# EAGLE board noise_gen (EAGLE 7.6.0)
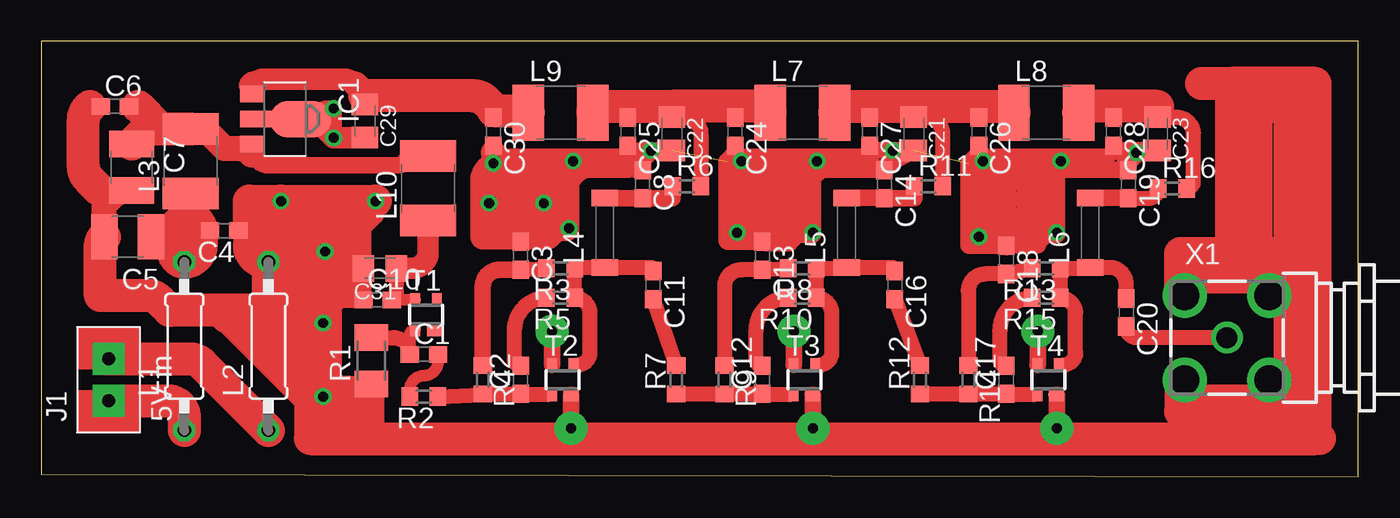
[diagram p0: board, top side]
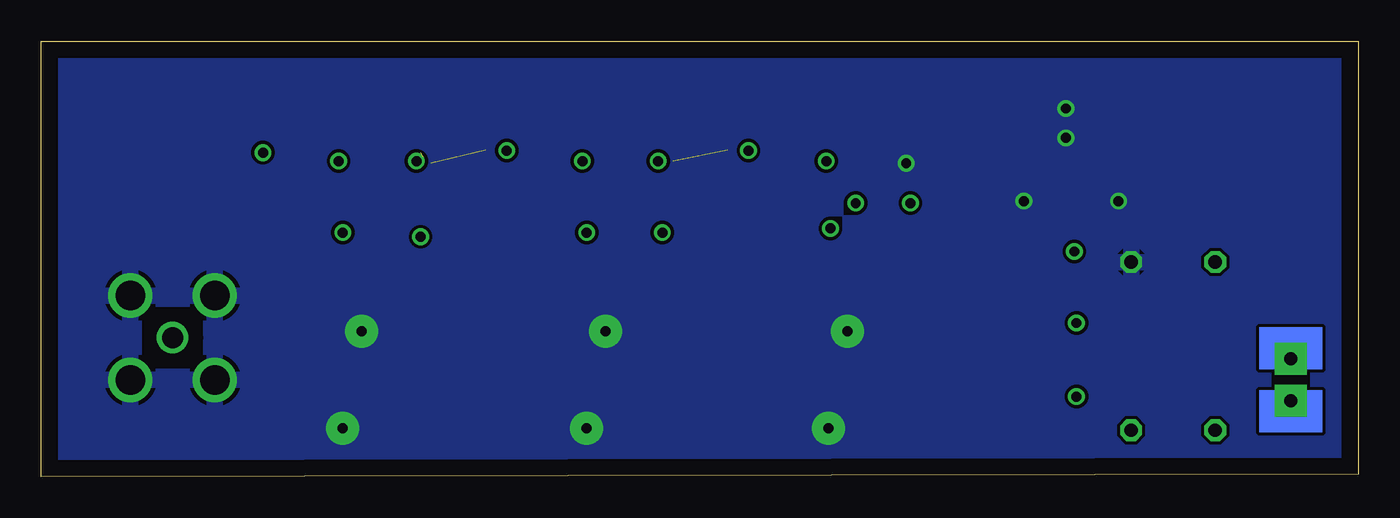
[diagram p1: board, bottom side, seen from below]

Size 79.55 x 26.28 mm. Coordinates in mm from the lower left corner, seen from the top.
Outline: 0,0.13 79.55,0 79.55,26.28 0,26.28 0,0.13
Copper layers (1*16): Top 0.035mm / dielectric 1.5mm / Bottom 0.035mm
Design rules "default": minimum track width 10mil, minimum drill 24mil, track to track 8mil, track to pad 8mil, pad to pad 8mil, via to via 8mil, smd to smd 8mil, copper to edge 40mil, drill to drill 8mil, minimum pad ring 10mil, minimum via ring 8mil, stop-mask expansion 4mil, vias tented up to drill 0mil, thermal gap 10mil

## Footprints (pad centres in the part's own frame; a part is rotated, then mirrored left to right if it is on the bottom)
C0603 = smd 1.1 x 1: 1 -0.85,0; 2 0.85,0
C1210 = smd 1.6 x 2.7: 1 -1.4,0; 2 1.4,0
C0805K = smd 1.3 x 1.6: 1 -1,0; 2 1,0
SOT89 = smd 1 x 1.5: 1 -1.499,-1.981; 3 1.499,-1.981 | smd 1 x 2: 2 0,-1.727 | smd 2.2 x 3.7: 2@1 0,0.94
H2-2.54_BIIG = drill 0.8 pad 1.93 square: 1 0,0; 2 0,2.54
0207/10 = drill 0.813 octagon: 1 -5.08,0; 2 5.08,0
L1812 = smd 1.9 x 3.4: 1 -1.95,0; 2 1.95,0
L4516C = smd 1 x 1.6: 1 -2.1,0; 2 2.1,0
M1206 = smd 1.6 x 2: 1 -1.4,0; 2 1.4,0
R0603 = smd 1 x 1.1: 1 -0.85,0; 2 0.85,0
SOT343R = smd 0.9 x 0.8: 1 0.5,-0.9 | smd 0.6 x 0.8: 2 -0.65,-0.9; 3 -0.65,0.9; 4 0.65,0.9
BU-SMA-G = drill 1.27: 1 0,0 | drill 1.778: 2 -2.55,2.55; 3 2.55,2.55; 4 2.55,-2.55; 5 -2.55,-2.55

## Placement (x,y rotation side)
C1  1n  [C0603]  23.11,7.37 0 top
C2  1n  [C0603]  28.96,5.84 90 top
C3  1n  [C0603]  28.96,13.34 270 top
C4  1 nF  [C0603]  11.05,14.86 180 top
C5  10 uF  [C1210]  5.21,14.48 180 top
C6  1 nF  [C0603]  4.45,22.35 0 top
C7  10 uF  [C1210]  5.46,18.67 270 top
C8  3n3  [C0603]  36.32,17.65 270 top
C10  3n3  [C0603]  20.32,10.67 0 top
C11  1n  [C0603]  36.96,11.56 270 top
C12  1n  [C0603]  43.56,5.84 90 top
C13  1n  [C0603]  43.56,13.34 270 top
C14  3n3  [C0603]  50.93,17.65 270 top
C16  1n  [C0603]  51.56,11.56 270 top
C17  1n  [C0603]  58.29,5.84 90 top
C18  1n  [C0603]  58.29,13.08 270 top
C19  3n3  [C0603]  65.66,17.65 270 top
C20  [C0603]  65.53,9.91 270 top
C21  100nF  [C0805K]  52.7,20.7 270 top
C22  100nF  [C0805K]  38.1,20.7 270 top
C23  100nF  [C0805K]  67.44,20.7 270 top
C24  1 nF  [C0603]  41.91,20.83 270 top
C25  1 nF  [C0603]  35.43,20.83 270 top
C26  1 nF  [C0603]  56.64,20.83 270 top
C27  1 nF  [C0603]  50.04,20.83 270 top
C28  1 nF  [C0603]  64.77,20.83 270 top
C29  100nF  [C0805K]  19.56,21.46 270 top
C30  1 nF  [C0603]  27.3,20.83 270 top
C31  100nF  [C0805K]  20.45,12.57 180 top
IC1  78L3.3F  [SOT89]  14.73,21.59 270 top
J1  5V in  [H2-2.54_BIIG]  4.06,4.57 0 top
L1  [0207/10]  8.64,7.87 90 top
L2  [0207/10]  13.72,7.87 90 top
L3  [L1812]  9.02,19.05 90 top
L4  60 nH  [L4516C]  34.04,14.73 90 top
L5  60 nH  [L4516C]  48.64,14.73 90 top
L6  60 nH  [L4516C]  63.37,14.73 90 top
L7  [L1812]  45.97,21.97 0 top
L8  [L1812]  60.71,21.97 0 top
L9  [L1812]  31.37,21.97 0 top
L10  [L1812]  23.37,17.4 90 top
R1  1k5  [M1206]  19.94,6.98 90 top
R2  18  [R0603]  23.11,4.83 180 top
R3  1k5  [R0603]  31.37,12.57 180 top
R4  1k5  [R0603]  26.67,5.84 270 top
R5  510R  [R0603]  31.37,10.79 180 top
R6  100  [R0603]  38.99,17.53 0 top
R7  18  [R0603]  38.35,5.84 90 top
R8  1k5  [R0603]  45.97,12.57 180 top
R9  1k5  [R0603]  41.27,5.84 270 top
R10  510R  [R0603]  45.97,10.79 180 top
R11  100  [R0603]  53.59,17.53 0 top
R12  18  [R0603]  53.09,5.84 90 top
R13  1k5  [R0603]  60.71,12.57 180 top
R14  1k5  [R0603]  56.01,5.84 270 top
R15  510R  [R0603]  60.71,10.79 180 top
R16  100  [R0603]  68.33,17.4 0 top
T1  BFG425W  [SOT343R]  23.24,9.78 0 top
T2  BFG425W  [SOT343R]  31.5,5.84 0 top
T3  BFG425W  [SOT343R]  46.1,5.84 0 top
T4  BFG425W  [SOT343R]  60.83,5.84 0 top
X1  BU-SMA-G  [BU-SMA-G]  71.63,8.38 0 top

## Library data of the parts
C1-C8 C10-C14 C16-C31 L1-L10 R1-R16 = rcl
IC1 = linear
J1 = Seeed-OPL-Connector
T1-T4 = mylib
X1 = con-coax; OC_FARNELL: unknown; OC_NEWARK: unknown

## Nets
GND: C3.1 C4.1 C5.2 C6.1 C7.2 C8.1 C10.1 C13.1 C14.1 C18.1 C19.1 C21.2 C22.2 C23.2 C24.2 C25.2 C26.2 C27.2 C28.2 C29.2 C30.2 C31.2 IC1.2 IC1.2@1 L2.2 R1.1 T2.1 T2.3 T3.1 T3.3 T4.1 T4.3 X1.2 X1.3 X1.4 X1.5
N$1: C29.1 C30.1 IC1.1 L9.1
N$2: C1.2 R2.2
N$3: C2.1 R2.1 R4.2 T2.2
N$4: C3.2 R3.2 R4.1
N$5: C2.2 R5.2
N$6: C11.1 L4.1 R3.1 R5.1 T2.4
N$7: J1.1 L1.1
N$8: C4.2 C5.1 L1.2 L3.1
N$9: J1.2 L2.1
N$10: C6.2 C7.1 IC1.3 L3.2 L10.2
N$11: C8.2 L4.2 R6.1
N$12: C1.1 R1.2 T1.2
N$13: C10.2 C31.1 L10.1 T1.3
N$14: C11.2 R7.2
N$15: C12.1 R7.1 R9.2 T3.2
N$16: C13.2 R8.2 R9.1
N$17: C12.2 R10.2
N$19: C14.2 L5.2 R11.1
N$20: C16.2 R12.2
N$21: C17.1 R12.1 R14.2 T4.2
N$22: C18.2 R13.2 R14.1
N$23: C17.2 R15.2
N$24: C20.1 L6.1 R13.1 R15.1 T4.4
N$25: C19.2 L6.2 R16.1
N$27: C16.1 L5.1 R8.1 R10.1 T3.4
N$28: C20.2 X1.1
N$32: C22.1 C24.1 C25.1 L7.1 L9.2 R6.2
N$34: C21.1 C26.1 C27.1 L7.2 L8.1 R11.2
N$35: C23.1 C28.1 L8.2 R16.2

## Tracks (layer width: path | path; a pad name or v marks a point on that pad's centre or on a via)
GND  (via drill 0.6 pad 1, 0.6 pad 2)  (3 unrouted)
  Top 0.406: T2.1
  Top 0.9: C6.1 2.92,22.35 | C19.1 65.66,18.54 65.66,18.92 | C28.2 64.77,19.68 64.77,19.56 | 50.04,19.68 50.04,19.56 | C26.2 56.64,19.56 | C24.2 41.91,19.56 | C25.2 35.43,19.56 | C8.1 36.32,18.92 | C30.2 27.3,19.56 | C31.2 arc-90 19.47,12.55 C10.1 | IC1.2 IC1.2@1 | C4.1 12.57,14.86
  Top 1: T2.3 30.86,6.74 v30.86,8.76 | T2.1 v32,2.92 | T3.3 arc90 45.47,6.76 v45.47,8.76 | T3.1 arc-90 T3.1 v46.61,2.92 | T4.3 arc90 60.2,6.76 v60.2,8.76 | T4.1 arc-90 61.34,4.93 v61.34,2.92 | 36.32,18.92 arc-90 35.43,19.81 C25.2 | C14.1 arc-90 50.04,19.39 50.04,19.68 | 50.04,19.68 C27.2 arc90 50.31,19.7 C21.2 50.55,18.54 | 35.56,19.68 C22.2 37.32,19.7 arc90 36.32,18.7 C8.1 36.14,18.5 arc-45 35.43,18.8 | 65.66,18.92 66.14,19.41 arc-45 66.85,19.7 C23.2 65.44,19.7 arc-45 C28.2 65.37,19.38 arc-45 65.66,18.67 65.66,18.54 | 35.43,18.8 | C3.1 28.96,14.48 | C10.1 18.03,10.67 17.65,10.29 17.65,5.97 18.04,5.58 R1.1 | C31.2 19.43,12.59 19.43,14.99 20.19,15.75 v20.19,16.64 | 11.39,9.56 11.86,10.03 12.45,10.03 | 41.91,19.56 41.66,19.3 | 41.66,19.3 41.4,19.05 41.4,14.22 41.44,14.19 C13.1 | 56.64,19.56 56.01,18.92 56.01,13.97 56.05,13.93 C18.1 | 74.68,13.46 74.55,13.46 74.3,13.72 73.41,13.72 | 75.44,3.43 74.93,3.94 74.55,3.94 | 64.77,19.68 64.39,19.3 56.52,19.3 | 50.04,19.68 49.66,19.3 41.66,19.3 | 16.76,21.84 17.14,22.22 v17.65,22.22 v17.65,20.45
  Top 1.3: C29.2 17.69,20.46 arc45 v17.65,20.45 16.8,21.3 arc45 16.1,21.59 IC1.2@1
  Top 1.5: C5.2 arc45 C5.2 3.81,16.38 4.4,16.98 arc-45 5.11,17.27 C7.2 arc45 C7.2 3.56,17.27 | 27.3,19.56 v27.3,18.92 26.96,18.58 arc45 26.67,17.87 26.67,14.48 28.96,14.48 30.61,14.48 30.82,14.69 arc-45 31.53,14.99 31.75,14.99 31.75,17.91 32.35,18.5 arc-45 33.05,18.8 35.43,18.8
  Top 2: 3.56,17.27 2.83,17.99 arc-45 2.54,18.7 2.54,21.56 arc-45 2.83,22.26 2.92,22.35 | C5.2 arc45 3.56,13.87 3.56,10.92 6.44,10.92 arc-45 7.15,10.63 7.75,10.03 12.45,10.03 12.72,10.03 arc90 13.72,11.03 L2.2 13.57,12.95 arc-90 12.57,13.95 12.57,14.86 12.57,16.64 v14.48,16.64 v20.19,16.64 | 11.18,9.65 arc-45 11.39,9.56 16.26,4.7 16.26,2.29 32,2.29 | 32,2.29 v32,2.92 | X1.2 68.83,11.18 68.83,13.46 74.55,13.46 74.55,11.3 X1.3 | X1.5 68.83,5.59 68.83,3.94 74.55,3.94 74.55,5.46 X1.4 | 32,2.29 46.61,2.29 | 46.61,2.29 v46.61,2.92 | 46.61,2.29 61.34,2.29 | 61.34,2.29 v61.34,2.92 | 61.34,2.29 76.96,2.29 | 77.22,2.29 76.96,2.29 | 76.96,2.29 76.96,23.75 71.88,23.75 | 70.1,23.75 71.88,23.75 | 71.88,23.75 71.88,13.72 73.41,13.72 73.41,22.35 75.31,22.35 75.31,22.22 75.44,22.22 75.44,3.43
  pour Bottom: -1.27,-1.14 -1.27,26.8 81.28,26.8 81.28,-1.14
N$1
  Top 0.9: 27.3,22.1 C30.1 27.3,22.22 | 12.7,23.49 12.7,23.14 arc90 IC1.1 12.75,23.5 arc45 12.7,23.62 | C29.1 19.56,22.99 19.56,23.11
  Top 1.3: 18.96,23.71 arc45 18.25,24 13.49,24 arc45 12.79,23.71
  Top 1.5: 19.56,23.11 18.96,23.71 | 12.79,23.71 12.7,23.62
  Top 2: 27.3,22.1 29.11,22.1 arc-45 L9.1 | 27.3,22.22 26.84,22.69 arc45 26.13,22.99 19.56,22.99
N$2
  Top 0.7: C1.2 23.96,6.95 arc-90 23.11,6.1 arc90 22.26,5.25 R2.2
N$3
  Top 0.1: 26.63,4.95 arc90 R4.2
  Top 0.6: T2.2 30.62,4.94 arc-90 30.61,4.95
  Top 0.9: R2.1 26.63,4.95 arc90 R4.2 C2.1 arc90 29,4.95 30.61,4.95
N$4
  Top 0.9: C3.2 R3.2
  Top 1: C3.2 27.67,12.49 arc90 26.67,11.49 R4.1
N$5
  Top 0.9: R5.2 arc90 28.57,8.85 28.57,7.07 arc90 C2.2
N$6
  Top 0.6: T2.4 32.37,6.74 arc-90 32.38,6.73
  Top 0.9: 32.38,6.73 arc90 33.15,7.49 33.15,9.87 arc90 R5.1 R3.1 arc-90 32.28,12.63 L4.1 36.73,12.63 arc-90 C11.1
N$7
  Top 2: J1.1 7.64,4.57 arc-90 8.64,3.57 L1.1
N$8
  Top 0.9: C4.2 9.65,14.86
  Top 1.5: C5.1 6.7,14.48 arc45 7.41,14.77 8.72,16.09 arc45 9.02,16.8 L3.1
  Top 2: 8.72,16.09 9.44,15.38 arc-45 9.65,14.86 9.65,13.95 arc-90 8.65,12.95 L1.2 arc-90 8,13.59 8,14.22
N$9
  Top 2: J1.2 8.98,7.11 arc-45 9.69,6.82 L2.1
N$10
  Top 0.9: C6.2 5.84,22.35 | IC1.3 arc90 12.7,20.04 12.7,19.43
  Top 1: L10.2 22.68,19.35 arc45 21.98,19.06 21.72,18.8 13.75,18.8 arc-45 13.04,19.09 12.7,19.43
  Top 1.5: L3.2 9.45,21 arc-45 10.15,20.71 11.05,19.81 11.9,19.81 arc-45 12.61,19.52 12.7,19.43
  Top 2: C7.1 6.1,20.71 arc-45 6.81,21 7.37,21 | 7.37,21 L3.2 | 5.84,22.35 7.07,21.12 arc45 7.37,21
N$11
  Top 1: L4.2 34.06,16.8 C8.2 38.14,16.8 R6.1
N$12
  Top 0.7: T1.2 arc90 22.26,8.55 C1.1
  Top 0.9: R1.2 21.26,8.38 arc-90 22.26,7.38 C1.1
N$13
  Top 0.7: T1.3 21.18,10.68 arc90 C10.2
  Top 0.9: C10.2 arc90 21.45,10.95 C31.1
  Top 1.3: C31.1 22.37,12.57 arc90 23.37,13.57 L10.1
N$14
  Top 0.9: C11.2 R7.2
N$15
  Top 0.6: T3.2 45.22,4.94 arc-90 45.21,4.95
  Top 0.9: R7.1 R9.2 C12.1 arc90 43.6,4.95 45.21,4.95
N$16
  Top 0.9: R9.1 41.27,11.49 arc-90 42.27,12.49 C13.2 R8.2
N$17
  Top 0.9: R10.2 arc90 43.18,8.85 43.18,7.07 arc90 C12.2
N$18  (via drill 0.6 pad 1)
  Top 1.5: 35.43,19.05 v32.13,19.05 27.43,19.05
N$19
  Top 1: L5.2 50.93,16.83 C14.2 52.74,16.8 R11.1
N$20
  Top 0.9: C16.2 R12.2
N$21
  Top 0.6: T4.2 59.95,4.94 arc-90 59.94,4.95
  Top 0.9: R12.1 R14.2 C17.1 arc90 58.33,4.95 59.94,4.95
N$22
  Top 0.9: R14.1 56.01,11.23 arc-90 57.01,12.23 C18.2 R13.2
N$23
  Top 0.9: R15.2 arc90 57.91,8.85 57.91,7.07 arc90 C17.2
N$24
  Top 0.6: T4.4 61.71,6.74 arc-90 61.72,6.73
  Top 0.9: 61.72,6.73 arc90 62.48,7.49 62.48,9.87 arc90 R15.1 R13.1 63.31,12.57 arc90 L6.1 64.53,12.63 arc-90 65.53,11.63 C20.1
N$25
  Top 0.9: C19.2 66.88,16.8 arc90 R16.1
  Top 1: L6.2 65.66,16.83 C19.2
N$26  (via drill 0.6 pad 1)
  Top 1: 58.29,13.84 58.42,13.97 60.07,13.97 | 60.07,13.97 60.2,13.97 | 60.07,13.97 60.71,14.61 61.34,14.61 v61.34,14.73 61.34,18.16 61.72,18.54 65.41,18.54
N$27
  Top 0.6: T3.4 46.98,6.74 arc-90 46.99,6.73
  Top 0.9: 46.99,6.73 arc90 47.75,7.49 47.75,9.87 arc90 R10.1 R8.1 48.58,12.57 arc90 L5.1 51.34,12.63 arc-90 C16.1
N$28
  Top 0.9: X1.1 66.21,8.38 arc-90 C20.2
N$29
  Top 1.5: 19.94,5.46 19.94,2.54
N$30
  Top 1.5: 18.92,15.62 18.41,15.62 18.41,11.3 16.76,11.3 16.76,4.57
N$31
  Top 1.5: 17.14,5.33 18.54,5.33 18.54,3.43 17.4,3.43 17.4,4.19
N$32
  Top 0.9: C22.1 38.84,21.7 arc-90 39.84,20.7 R6.2 | C25.1 35.43,22.1 | C24.1 41.91,22.1
  Top 1: 35.43,22.1 35.43,22.22 arc90 35.31,22.35 | 41.91,22.1 arc90 41.66,22.35
  Top 1.3: C22.1 38.1,22.35
  Top 2: L9.2 arc-90 33.7,22.35 35.31,22.35 38.1,22.35 41.66,22.35 43.64,22.35 arc-90 L7.1
N$33  (via drill 0.6 pad 1)
  Top 2: 13.72,8.38 14.1,8.38 14.1,15.24 17.02,15.24 17.02,15.11 17.14,15.11 v17.14,13.59 17.14,12.32 15.75,12.32 15.75,7.24
N$34
  Top 0.9: C21.1 53.44,21.7 arc-90 54.44,20.7 R11.2 | C27.1 50.04,22.1 | C26.1 56.64,22.1
  Top 1: 56.64,22.1 56.9,22.35 | 50.04,22.1 50.55,22.35 | C21.1 53.09,22.35
  Top 2: L7.2 48.01,22.06 arc-45 48.72,22.35 50.55,22.35 53.09,22.35 56.9,22.35 58.17,22.35 arc-45 58.52,22.2 L8.1
N$35
  Top 0.9: R16.2 arc90 69.6,17.82 69.6,20.7 arc90 68.6,21.7 C23.1 | C28.1 64.77,22.1
  Top 1: 64.77,22.1 64.52,22.35
  Top 1.3: C23.1 67.44,22.35
  Top 2: 67.44,22.35 64.52,22.35 63.45,22.35 arc45 62.74,22.06 L8.2
N$36
  Top 2: 15.62,14.86 15.62,12.57
N$37
  Top 2: 27.56,17.65 30.99,17.65 30.99,16 28.07,16 28.07,15.75
N$38  (via drill 0.6 pad 1)
  other vias: 17.02,4.83
N$39  (via drill 0.6 pad 1)
  other vias: 17.02,9.27
N$40  (via drill 0.6 pad 1)
  other vias: 27.05,16.51
N$41  (via drill 0.6 pad 1)
  other vias: 30.35,16.51
N$42  (via drill 0.6 pad 1)
  other vias: 31.88,14.99
N$43
  Top 2: 68.96,12.07 74.42,12.07
N$44
  Top 2: 69.6,4.57 75.31,4.57 75.31,4.7
N$45  (via drill 0.6 pad 1)
  Top 1: 43.69,14.22 43.81,14.1 45.21,14.1 45.72,14.61 46.61,14.61 v46.61,14.73 46.61,18.03 47.12,18.54 50.93,18.54
N$46
  Top 2: 45.97,18.67 45.59,18.29 42.29,18.29 42.55,18.03 42.55,15.11 42.93,15.49 45.21,15.49 45.34,15.62 45.34,16.89 44.07,16.89
N$47
  Top 2: 56.9,18.16 57.02,18.29 60.45,18.29 59.94,17.78 59.94,15.49 59.69,15.24 56.9,15.24 57.15,15.49 57.15,16.76 58.04,16.76
N$48  (via drill 0.6 pad 1)
  other vias: 46.86,19.05
N$49  (via drill 0.6 pad 1)
  other vias: 42.29,19.05
N$50  (via drill 0.6 pad 1)
  other vias: 56.9,19.05
N$51  (via drill 0.6 pad 1)
  other vias: 61.59,19.05
N$52  (via drill 0.6 pad 1)
  other vias: 42.04,14.73
N$53  (via drill 0.6 pad 1)
  other vias: 56.64,14.48
N$54  (via drill 0.6 pad 1)
  other vias: 66.17,19.56
N$55  (via drill 0.6 pad 1)
  other vias: 51.44,19.68
N$56  (via drill 0.6 pad 1)
  other vias: 36.83,19.68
